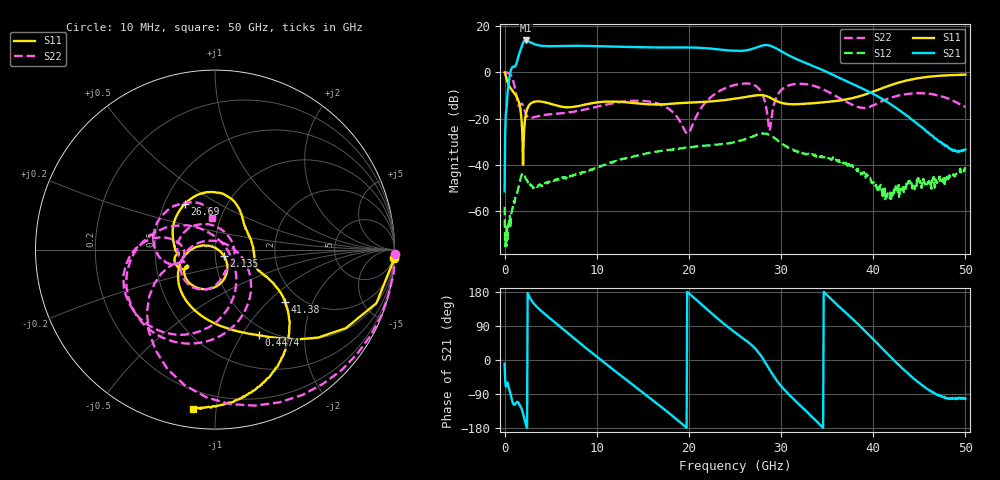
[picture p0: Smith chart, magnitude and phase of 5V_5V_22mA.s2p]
! MARKI MICROWAVE INC.
! Date:  1/07/2020
! Model Number:  APM-6849CH
! Description:  2-port Small Signal S-parameter data for APM-6849CH
! Frequency Range:  10 MHz to 50 GHz
! Port Configuration:  PORT 1: Input
!  PORT 2: Output
! Bias Condition: Vc = +5V, Vb = +5V
! APM-6849CH s2p files are only valid for small signal conditions (below -5 dBm input power)
!S2P File: Measurements: Mag<S11> Ang<S11>, Mag<S21> Ang<S21>, Mag<S12> Ang<S12>, Mag<S22> Ang<S22>!row 1
# Hz S  dB  R 50
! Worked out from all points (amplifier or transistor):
!   801 points, 10 MHz to 50 GHz, reference 50 ohm
!   highest |S21| = 13.8 dB at 2.322 GHz (marker M1)
!   |S21| within 3 dB of that: 1.833 GHz to 16.07 GHz (14.23 GHz wide, 159 % of centre)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
!   unconditionally stable (mu >= 1): 118.2 MHz to end of sweep
!   at 8.321 GHz: K = 18.99, MAG = 11.7 dB, |S12| = -43.6 dB
!   at 25 GHz: K = 3.68, MAG = 11.1 dB, |S12| = -30.2 dB
!   at 50 GHz: K = 558.32, MAG = -26.2 dB, |S12| = -41.9 dB
!   S11 on the Smith chart (normalised r, x): 10 MHz: -1, -41; 447.4 MHz: 0.89, -1.19; 2.135 GHz: 1.10, -0.07; 26.69 GHz: 0.64, +0.36; 41.38 GHz: 1.67, -1.28; 50 GHz: 0.10, -0.87
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1e7  0.01 -2.8  -51.44 -9.9  -58.11 105.6  0.04 -1.3
4.474125e8  -5.43 -63.0  -4.74 -71.0  -65.17 -3.9  -0.36 -51.2
1.5097e9  -12.26 -147.6  6.94 -112.8  -49.93 -70.3  -14.37 -159.7
2.134575e9  -24.46 -34.0  13.53 -153.7  -44.76 -146.4  -15.93 116.7
2.322038e9  -17.87 -57.2  13.80 -170.3  -46.32 -163.4  -18.07 83.2
3.071888e9  -12.91 -102.4  12.46 152.2  -49.95 -175.4  -19.54 5.1
4.571588e9  -13.09 -139.7  11.34 117.2  -47.46 178.7  -18.26 -40.1
8.383325e9  -14.22 -146.5  11.47 40.6  -43.14 133.2  -16.36 -73.2
1.175765e10  -12.60 -163.2  11.16 -24.7  -38.94 97.6  -13.32 -96.6
1.431964e10  -13.38 -173.2  10.93 -73.1  -36.02 62.7  -12.24 -123.3
1.669416e10  -13.89 -174.2  10.79 -118.0  -34.15 27.2  -13.59 -155.3
2.038092e10  -13.02 178.1  10.72 168.0  -32.32 -30.1  -22.83 22.6
2.269296e10  -12.45 167.4  10.17 118.4  -31.36 -70.9  -9.70 -53.4
2.5005e10  -11.36 148.8  9.31 72.8  -30.15 -114.2  -5.42 -102.5
2.669216e10  -10.32 123.3  9.94 41.6  -28.08 -155.4  -5.00 -144.6
2.825435e10  -10.02 82.6  11.80 -4.8  -26.50 144.9  -12.81 143.9
2.956659e10  -12.46 50.6  10.18 -55.3  -29.08 90.3  -10.20 -73.3
3.337832e10  -13.37 -0.7  2.86 -150.4  -35.39 15.4  -5.64 -165.8
3.644021e10  -12.10 -23.2  -2.62 137.9  -38.81 -53.5  -11.36 166.3
4.137672e10  -6.24 -36.7  -12.45 20.4  -53.51 136.4  -11.74 -161.9
4.168916e10  -5.81 -38.7  -13.22 13.0  -53.14 114.8  -11.30 -163.8
5e10  -0.96 -97.9  -33.33 -101.6  -41.92 -65.1  -14.98 94.7
